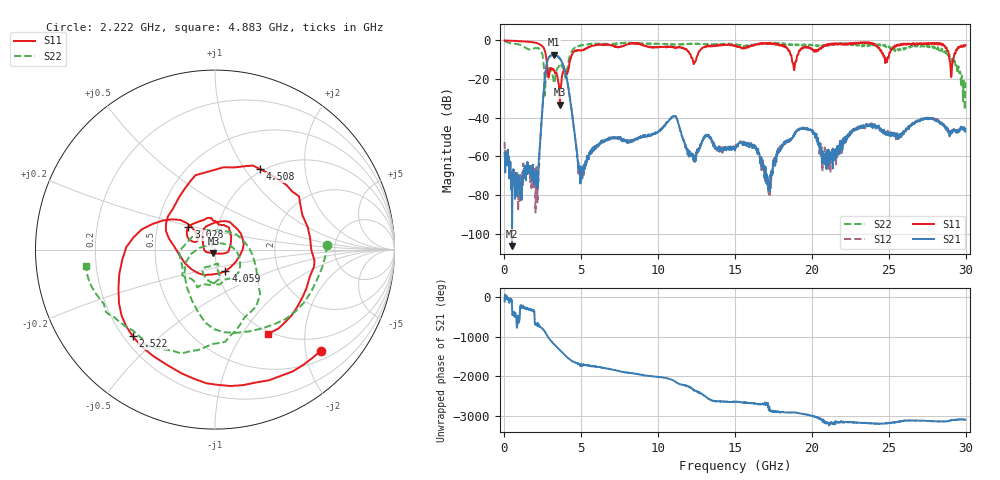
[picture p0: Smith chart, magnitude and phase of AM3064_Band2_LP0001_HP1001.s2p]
# Hz S DB R 50.0
!freq dBS11 angS11 dBS21 angS21 dBS12 angS12 dBS22 angS22
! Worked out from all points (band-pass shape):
!   1600 points, 10 MHz to 29.98 GHz, reference 50 ohm
!   highest |S21| = -7.38 dB at 3.215 GHz (marker M1); lowest = -106.5 dB at 497.3 MHz (marker M2)
!   |S21| within 3 dB of the highest: 2.805 GHz to 3.682 GHz (876.3 MHz wide, 27 % of centre)
!   lowest |S11| = -33.3 dB at 3.609 GHz (marker M3), VSWR 1.04, Z = 49.1 - j1.96 ohm
!   |S11| at or under -10 dB: 2.735 GHz to 4.277 GHz (1.541 GHz wide, 44 % of centre); 18.7 GHz to 19 GHz (297.2 MHz wide, 1.58 % of centre); 28.95 GHz to 29.2 GHz (254.7 MHz wide, 0.876 % of centre)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
!   |S22| runs from -36.0 to -0.2 dB; largest |S21 - S12| = 0.014
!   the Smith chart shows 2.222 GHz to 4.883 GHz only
!   S11 on the Smith chart (normalised r, x): 2.222 GHz: 0.69, -2.32; 2.522 GHz: 0.24, -0.41; 3.028 GHz: 0.72, +0.19; 4.059 GHz: 1.09, -0.27; 4.508 GHz: 0.97, +1.18; 4.883 GHz: 0.97, -1.31
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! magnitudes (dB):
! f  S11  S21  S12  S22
! 10 MHz  0.0  -58.1  -52.5  -0.2
! 497.3 MHz  -0.2  -106.5  -82.8  -1.5
! 2.222 GHz  -1.8  -64.6  -65.8  -4.1
! 2.522 GHz  -3.5  -29.6  -29.6  -10.2
! 3.028 GHz  -14.3  -7.8  -7.8  -15.1
! 3.215 GHz  -15.2  -7.4  -7.6  -21.7
! 3.609 GHz  -33.3  -9.6  -9.3  -13.0
! 4.059 GHz  -17.5  -19.8  -19.9  -16.0
! 4.508 GHz  -5.8  -44.8  -44.5  -4.3
! 4.883 GHz  -5.1  -67.8  -64.4  -2.8
! 5.015 GHz  -5.2  -71.5  -68.5  -2.6
! 6.327 GHz  -2.3  -52.2  -52.5  -1.8
! 10 GHz  -3.5  -47.4  -47.1  -1.8
! 15 GHz  -2.7  -55.7  -55.0  -1.9
! 16.35 GHz  -2.2  -55.3  -55.4  -2.3
! 17.18 GHz  -1.8  -72.5  -79.6  -1.6
! 18.06 GHz  -2.3  -55.5  -55.0  -1.8
! 19.99 GHz  -4.3  -46.9  -46.6  -2.1
! 21.06 GHz  -2.2  -64.4  -63.3  -1.9
! 25 GHz  -8.5  -48.5  -48.7  -3.0
! 28.56 GHz  -2.5  -43.4  -43.7  -5.0
! 29.98 GHz  -2.4  -45.9  -47.1  -21.7
